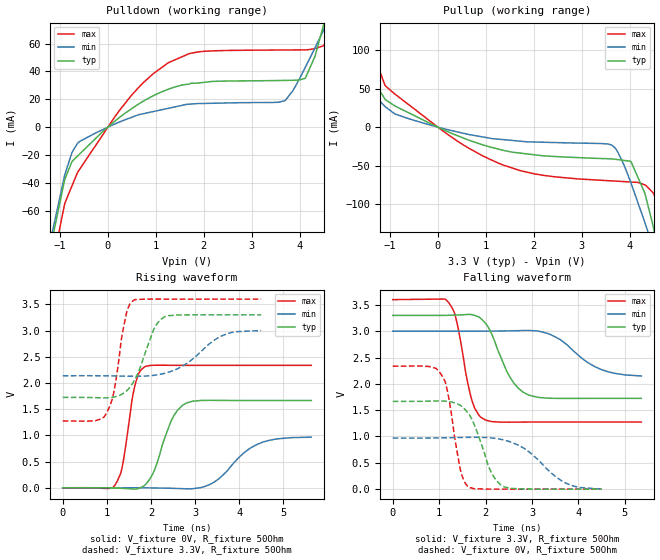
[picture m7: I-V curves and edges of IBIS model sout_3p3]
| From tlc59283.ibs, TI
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|   sout_3p3 Model
[Model]   sout_3p3
Model_type   Output
Polarity   Non-Inverting
Vmeas = 1.65
Vref = 1.65
Cref = 15pF
Rref = 50
|   typ   min   max
C_comp   1.280e-12   1.204e-12   1.424e-12
| Where nom  PVT is Nominal Process, 3.3V, 27C
|   Fast PVT is Strong Process,  3.6V, -40C
|   Slow PVT is Weak Process,   3V, 125C
[Voltage Range]   3.3   3   3.6
|Ambient Temperature   25   85   -40
|Junction Temperature
[Temperature Range]   27   125   -40
[Pullup Reference]   3.3   3   3.6
[Pulldown Reference]   0   0   0
[Power Clamp Reference]   3.3   3   3.6
[GND Clamp Reference]   0   0   0
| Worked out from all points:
|   slope of the pulldown table from 0 to 0.495 V, typ, clamps not added: 37.5 ohm
|   slope of the pullup table from 0 to 0.495 V, typ, clamps not added: 37.5 ohm
|   falling waveform, V_fixture 3.3V, R_fixture 50Ohm: 20-80 % time 479ps typ, 747ps min, 298ps max; typ from 3.3 V to 1.73 V
|   rising waveform, V_fixture 0V, R_fixture 50Ohm: 20-80 % time 415ps typ, 719ps min, 250ps max; typ from 0 V to 1.67 V
|   rising waveform, V_fixture 3.3V, R_fixture 50Ohm: 20-80 % time 428ps typ, 767ps min, 259ps max; typ from 1.73 V to 3.3 V
|   falling waveform, V_fixture 0V, R_fixture 50Ohm: 20-80 % time 416ps typ, 752ps min, 259ps max; typ from 1.67 V to 0 V
[Pulldown]
|   Voltage   I(typ)   I(min)   I(max)
-3.3V     -698.1mA   -507.8mA   -1.043A
-1.212V   -97.72mA   -84.24mA   -130.5mA
-1.084V   -68mA      -63.77mA   -86.29mA
-897.6mV  -37.4mA    -34.11mA   -54.73mA
-603mV    -19.78mA   -10.67mA   -31mA
633mV     16.46mA    8.838mA    28.18mA
1.706V    30.93mA    16.51mA    52.91mA
3.681V    33.53mA    18.87mA    55.36mA
4.115V    35.05mA    42.95mA    55.44mA
4.583V    85.14mA    75.84mA    64.22mA
4.68V     98.35mA    82.84mA    85.03mA
6.6V      352.2mA    220.4mA    597.4mA
[Pullup]
|   Voltage   I(typ)   I(min)   I(max)
-3.3V     319mA      181.6mA    601.6mA
-1.994V   148.1mA    88.67mA    296.7mA
-1.344V   63.02mA    42.38mA    111.9mA
-1.098V   35.91mA    26.48mA    53.72mA
-897mV    27.53mA    17.08mA    42.94mA
1.357V    -29.88mA   -16.15mA   -49.01mA
3.627V    -41.11mA   -23.29mA   -69.66mA
4.026V    -44.6mA    -72.42mA   -71.1mA
4.349V    -93.96mA   -129.9mA   -76.29mA
4.496V    -130.8mA   -157.6mA   -85.8mA
4.777V    -209.2mA   -213.6mA   -181mA
6.6V      -742.4mA   -593.4mA   -999.6mA
[Ramp]
R_load = 50
|   typ   min   max
dV/dt_r   0.999452/4.13107e-10   0.582339/7.19834e-10   1.40137/2.50108e-10
dV/dt_f   0.945142/4.77225e-10   0.517439/7.62971e-10   1.39473/2.97402e-10
[Falling Waveform]
V_fixture = 3.3V
V_fixture_min = 3V
V_fixture_max = 3.6V
R_fixture = 50Ohm
|   Time   V(typ)   V(min)   V(max)
0s        3.3V       3V         3.6V
1.21ns    3.303V     3V         3.538V
1.38ns    3.307V     3V         3.179V
1.715ns   3.312V     3V         1.662V
1.985ns   3.164V     3.001V     1.318V
2.525ns   2.129V     3.007V     1.272V
2.89ns    1.805V     3.015V     1.274V
3.59ns    1.724V     2.85V      1.275V
4.5ns     1.725V     2.27V      1.275V
5.355ns   1.725V     2.15V      1.275V
[Rising Waveform]
V_fixture = 0V
V_fixture_min = 0V
V_fixture_max = 0V
R_fixture = 50Ohm
|   Time   V(typ)   V(min)   V(max)
0s        1.217nV    7.603nV    889.5pV
1.185ns   -4.792mV   474uV      51.79mV
1.35ns    -10.75mV   540.1uV    402.9mV
1.65ns    -26.53mV   -6.706uV   1.994V
1.87ns    55.86mV    -1.549mV   2.312V
2.455ns   1.272V     -10.05mV   2.337V
2.8ns     1.615V     -19.22mV   2.336V
3.44ns    1.668V     112mV      2.336V
4.39ns    1.666V     821mV      2.336V
5.635ns   1.666V     966.2mV    2.336V
[Rising Waveform]
V_fixture = 3.3V
V_fixture_min = 3V
V_fixture_max = 3.6V
R_fixture = 50Ohm
|   Time   V(typ)   V(min)   V(max)
0s        1.725V     2.138V     1.276V
980ps     1.717V     2.136V     1.405V
1.16ns    1.732V     2.134V     1.83V
1.325ns   1.779V     2.131V     2.811V
1.445ns   1.846V     2.129V     3.331V
1.59ns    2.001V     2.128V     3.567V
2.055ns   3.008V     2.144V     3.601V
2.315ns   3.265V     2.185V     3.6V
3.63ns    3.3V       2.909V     3.6V
4.498ns   3.3V       2.999V     3.6V
[Falling Waveform]
V_fixture = 0V
V_fixture_min = 0V
V_fixture_max = 0V
R_fixture = 50Ohm
|   Time   V(typ)   V(min)   V(max)
0s        1.666V     970.6mV    2.336V
1.055ns   1.675V     974.1mV    2.164V
1.195ns   1.665V     976.2mV    1.79V
1.455ns   1.594V     980.9mV    378.4mV
1.645ns   1.42V      984.2mV    31.34mV
2.11ns    343.4mV    973.7mV    294.9uV
2.335ns   73.5mV     945mV      -574.3uV
2.825ns   3.674mV    777.1mV    -59.74uV
3.725ns   -143.4uV   116.7mV    13.9uV
4.495ns   21.38uV    1.912mV    6.271uV
